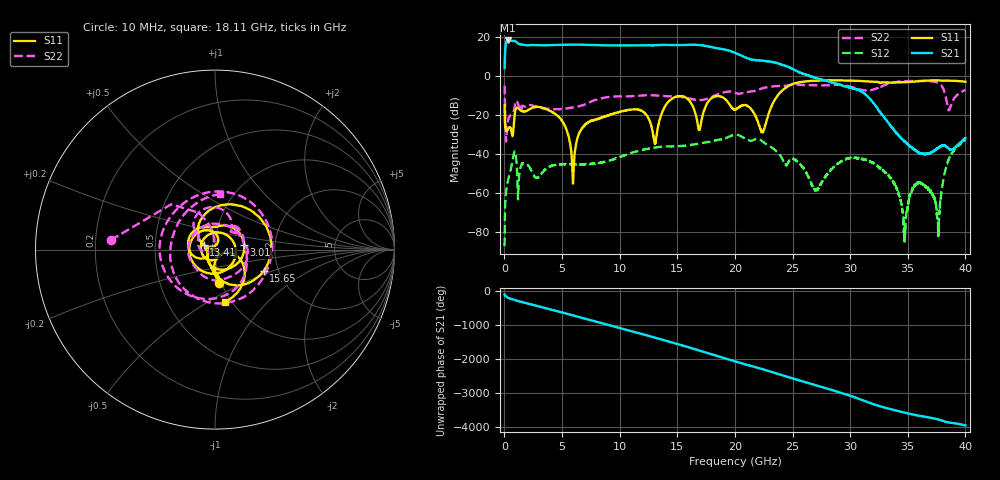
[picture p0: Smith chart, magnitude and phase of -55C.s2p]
#  HZ  S  DB  R  50.00
! Rohde & Schwarz Vector Network Analyzer
! Rohde-Schwarz,ZNB3032-4Port,1351505034101534,4.21
! Created: UTC 6/10/2026, 1:36:13 PM
! freq[Hz]  db:S11  ang:S11  db:S21  ang:S21  db:S12  ang:S12  db:S22  ang:S22
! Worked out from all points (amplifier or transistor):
!   3200 points, 10 MHz to 40 GHz, reference 50 ohm
!   highest |S21| = 18.5 dB at 285 MHz (marker M1)
!   |S21| within 3 dB of that: 88.35 MHz to 17.6 GHz (17.51 GHz wide, 198 % of centre)
!   unconditionally stable (mu >= 1): start of sweep to end of sweep
!   at 6.673 GHz: K = 13.27, MAG = 16.4 dB, |S12| = -45.1 dB
!   at 20.01 GHz: K = 3.37, MAG = 12.7 dB, |S12| = -29.8 dB
!   at 40 GHz: K = 287.72, MAG = -27.3 dB, |S12| = -32.2 dB
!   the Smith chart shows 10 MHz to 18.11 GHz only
!   S11 on the Smith chart (normalised r, x): 10 MHz: 0.97, -0.37; 3.01 GHz: 1.38, +0.07; 13.41 GHz: 0.88, +0.05; 15.65 GHz: 1.67, -0.44; 18.11 GHz: 0.93, -0.60
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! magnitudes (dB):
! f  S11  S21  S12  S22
! 10 MHz  -14.7  4.3  -87.1  -4.7
! 285 MHz  -27.2  18.5  -53.8  -22.8
! 847.6 MHz  -21.8  18.3  -38.8  -16.6
! 3.01 GHz  -15.7  16.1  -51.3  -15.6
! 5.035 GHz  -23.1  16.2  -45.0  -16.8
! 5.935 GHz  -53.1  16.3  -45.0  -15.9
! 6.685 GHz  -26.8  16.3  -45.1  -14.9
! 13.35 GHz  -24.9  16.1  -36.2  -9.8
! 13.41 GHz  -23.4  16.2  -36.2  -9.8
! 15.65 GHz  -10.6  16.2  -35.6  -10.8
! 16.9 GHz  -27.3  16.2  -34.4  -12.1
! 18.11 GHz  -10.5  14.9  -33.1  -10.2
! 20.01 GHz  -16.9  12.0  -29.8  -8.5
! 22.39 GHz  -28.2  8.1  -33.3  -6.1
! 26.67 GHz  -2.3  -0.1  -55.7  -4.5
! 30.05 GHz  -2.2  -5.8  -41.7  -5.3
! 33.34 GHz  -3.1  -24.0  -50.9  -3.7
! 34.72 GHz  -2.9  -33.3  -80.6  -2.4
! 35.92 GHz  -2.4  -39.0  -54.6  -2.3
! 37.61 GHz  -2.0  -36.8  -75.2  -3.3
! 38.49 GHz  -2.2  -36.7  -43.5  -16.0
! 40 GHz  -2.7  -31.6  -32.2  -6.9
